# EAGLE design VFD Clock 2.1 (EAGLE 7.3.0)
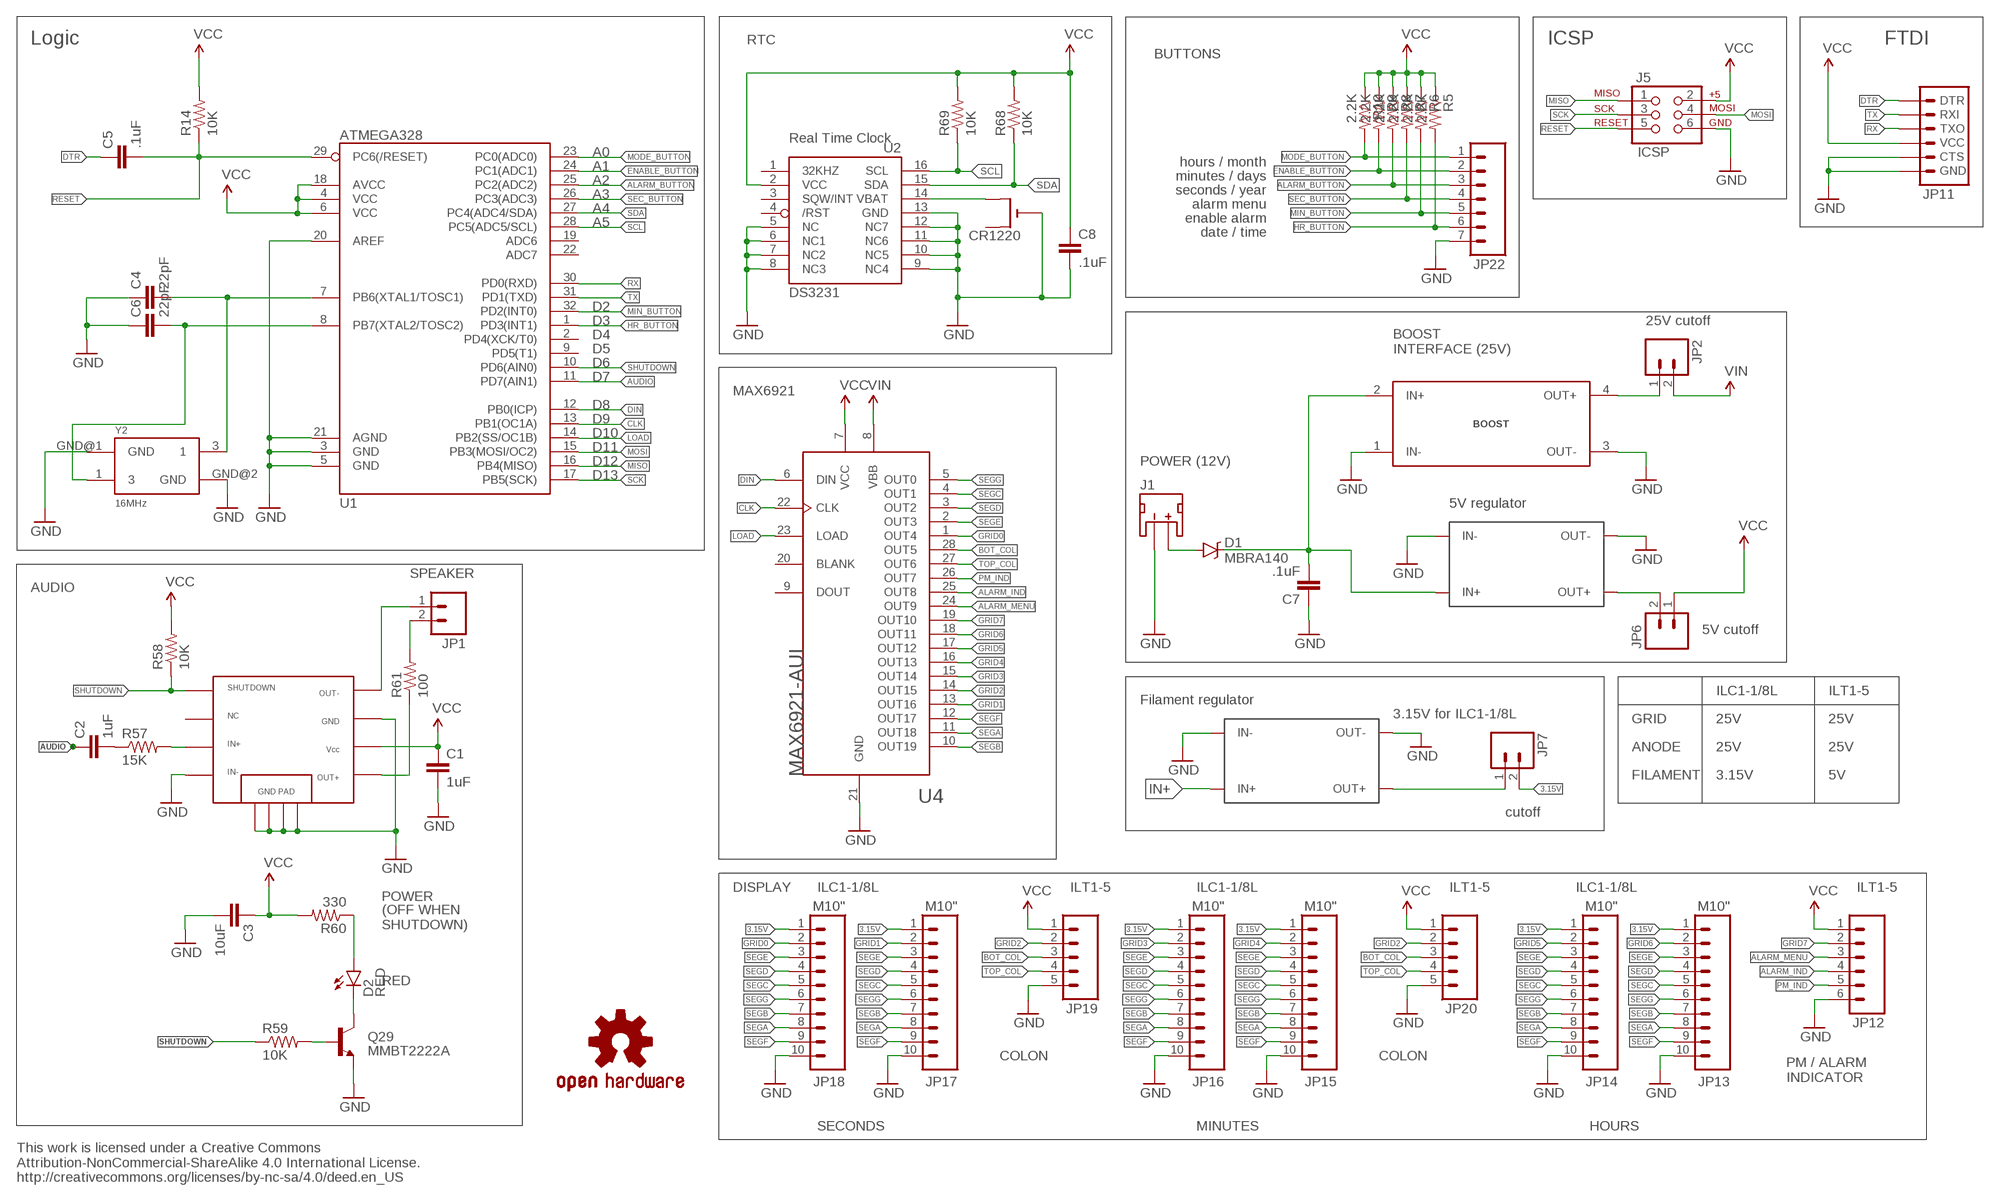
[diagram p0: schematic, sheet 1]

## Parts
3.15V  DCTODC  [DCTODC]
5V  DCTODC  [DCTODC]
C1  1uF  CAP0805  [0805]
C2  1uF  CAP0805  [0805]
C3  10uF  CAP0805  [0805]
C4  22pF  CAP0805  [0805]
C5  .1uF  CAP0805  [0805]
C6  22pF  CAP0805  [0805]
C7  .1uF  CAP0805  [0805]
C8  .1uF  CAP0805  [0805]
CR1220  CR1220SMT  [CR1220-SMD]
D1  MBRA140  [SMA-DIODE]
D2  RED  LED1206  [LED-1206]
J1  JST_2MM_MALE  [JST-2-SMD]
J5  ICSP  AVR_SPI_PRG_6PTH  [2X3]
JP1  M02PTH  [1X02]
JP2  M02PTH  [1X02]
JP6  M02PTH  [1X02]
JP7  M02PTH  [1X02]
JP11  ARDUINO_SERIAL_PROGRAMSMD  [1X06-SMD]
JP12  M06SIP  [1X06]
JP13  M10"  [1X10]
JP14  M10"  [1X10]
JP15  M10"  [1X10]
JP16  M10"  [1X10]
JP17  M10"  [1X10]
JP18  M10"  [1X10]
JP19  M05PTH  [1X05]
JP20  M05PTH  [1X05]
JP22  M07  [1X07]
Q29  MMBT2222A  TRANSISTOR_NPNSOT23-3  [SOT23-3]
R5  2.2K  RESISTOR0805-RES  [0805]
R6  2.2K  RESISTOR0805-RES  [0805]
R7  2.2K  RESISTOR0805-RES  [0805]
R8  2.2K  RESISTOR0805-RES  [0805]
R9  2.2K  RESISTOR0805-RES  [0805]
R10  2.2K  RESISTOR0805-RES  [0805]
R14  10K  RESISTOR0805-RES  [0805]
R57  15K  RESISTOR0805-RES  [0805]
R58  10K  RESISTOR0805-RES  [0805]
R59  10K  RESISTOR0805-RES  [0805]
R60  330  RESISTOR0805-RES  [0805]
R61  100  RESISTOR0805-RES  [0805]
R68  10K  RESISTOR0805-RES  [0805]
R69  10K  RESISTOR0805-RES  [0805]
U1  ATMEGA328  ATMEGA328_SMT  [TQFP32-08]
U2  DS3231  DS3231/SO  [SO16W]
U3  TPA2005  [MSOP8]
U4  MAX6921  [MAX6921]
U$2  BOOST  [BOOST]
U$7  OSHW-LOGOS  [OSHW-LOGO-S]
Y2  16MHz  OSCILLATOR5X3  [CRYSTAL-SMD-5X3]

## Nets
3.15V: JP7.2 JP13.1 JP14.1 JP15.1 JP16.1 JP17.1 JP18.1
5VOUT: 5V.OUT+ JP6.2
ALARM_BUTTON: JP22.3 R8.2 U1.25(PC2(ADC2))
ALARM_IND: JP12.4 U4.25(OUT8)
ALARM_MENU: JP12.3 U4.24(OUT9)
AUDIO: C2.1 U1.11(PD7(AIN1))
BOT_COL: JP19.3 JP20.3 U4.28(OUT5)
CLK: U1.13(PB1(OC1A)) U4.22(CLK)
DIN: U1.12(PB0(ICP)) U4.6(DIN)
DTR: C5.1 JP11.1(DTR)
ENABLE_BUTTON: JP22.2 R9.2 U1.24(PC1(ADC1))
FILAMENTOUT: 3.15V.OUT+ JP7.1
GND: 3.15V.IN- 3.15V.OUT- 5V.IN- 5V.OUT- C1.2 C3.2 C4.1 C6.1 C7.1 C8.2 CR1220.- J1.1(-) J5.6 JP11.5(CTS) JP11.6(GND) JP12.6 JP13.10 JP14.10 JP15.10 JP16.10 JP17.10 JP18.10 JP19.5 JP20.5 JP22.7 Q29.2(E) U1.3(GND) U1.5(GND) U1.20(AREF) U1.21(AGND) U2.5(NC) U2.6(NC1) U2.7(NC2) U2.8(NC3) U2.9(NC4) U2.10(NC5) U2.11(NC6) U2.12(NC7) U2.13(GND) U3.4 U3.7 U3.A U3.B U3.C U3.D U4.21(GND) U$2.1(IN-) U$2.3(OUT-) Y2.GND@1(GND) Y2.GND@2(GND)
GRID0: JP18.2 U4.1(OUT4)
GRID1: JP17.2 U4.13(OUT16)
GRID2: JP19.2 JP20.2 U4.14(OUT15)
GRID3: JP16.2 U4.15(OUT14)
GRID4: JP15.2 U4.16(OUT13)
GRID5: JP14.2 U4.17(OUT12)
GRID6: JP13.2 U4.18(OUT11)
GRID7: JP12.2 U4.19(OUT10)
HR_BUTTON: JP22.6 R5.2 U1.1(PD3(INT1))
IN+: 3.15V.IN+ 5V.IN+ C7.2 D1.C U$2.2(IN+)
IN+AMP: R57.2 U3.3
LOAD: U1.14(PB2(SS/OC1B)) U4.23(LOAD)
MIN_BUTTON: JP22.5 R6.2 U1.32(PD2(INT0))
MISO: J5.1 U1.16(PB4(MISO))
MODE_BUTTON: JP22.1 R10.2 U1.23(PC0(ADC0))
MOSI: J5.4 U1.15(PB3(MOSI/OC2))
N$1: JP2.1 U$2.4(OUT+)
N$7: CR1220.+$2(+1) U2.14(VBAT)
N$8: C6.2 U1.8(PB7(XTAL2/TOSC2)) Y2.1
N$28: JP1.2 R61.2
N$29: D2.A R60.1
N$30: C4.2 U1.7(PB6(XTAL1/TOSC1)) Y2.3
N$31: Q29.1(B) R59.2
N$33: D2.C Q29.3(C)
N$34: C2.2 R57.1
N$35: JP1.1 U3.8
N$36: R61.1 U3.5
N$39: D1.A J1.2(+)
PM_IND: JP12.5 U4.26(OUT7)
RESET: C5.2 J5.5 R14.1 U1.29(PC6(/RESET))
RX: JP11.3(TXO) U1.30(PD0(RXD))
SCK: J5.3 U1.17(PB5(SCK))
SCL: R69.1 U1.28(PC5(ADC5/SCL)) U2.16(SCL)
SDA: R68.1 U1.27(PC4(ADC4/SDA)) U2.15(SDA)
SEC_BUTTON: JP22.4 R7.2 U1.26(PC3(ADC3))
SEGA: JP13.8 JP14.8 JP15.8 JP16.8 JP17.8 JP18.8 U4.11(OUT18)
SEGB: JP13.7 JP14.7 JP15.7 JP16.7 JP17.7 JP18.7 U4.10(OUT19)
SEGC: JP13.5 JP14.5 JP15.5 JP16.5 JP17.5 JP18.5 U4.4(OUT1)
SEGD: JP13.4 JP14.4 JP15.4 JP16.4 JP17.4 JP18.4 U4.3(OUT2)
SEGE: JP13.3 JP14.3 JP15.3 JP16.3 JP17.3 JP18.3 U4.2(OUT3)
SEGF: JP13.9 JP14.9 JP15.9 JP16.9 JP17.9 JP18.9 U4.12(OUT17)
SEGG: JP13.6 JP14.6 JP15.6 JP16.6 JP17.6 JP18.6 U4.5(OUT0)
SHUTDOWN: R58.1 R59.1 U1.10(PD6(AIN0)) U3.1
TOP_COL: JP19.4 JP20.4 U4.27(OUT6)
TX: JP11.2(RXI) U1.31(PD1(TXD))
VCC: C1.1 C3.1 C8.1 J5.2 JP6.1 JP11.4(VCC) JP12.1 JP19.1 JP20.1 R5.1 R6.1 R7.1 R8.1 R9.1 R10.1 R14.2 R58.2 R60.2 R68.2 R69.2 U1.4(VCC) U1.6(VCC) U1.18(AVCC) U2.2(VCC) U3.6 U4.7(VCC)
VIN: JP2.2 U4.8(VBB)
Unconnected: CR1220.+$1(+) J1.NC1(PAD1) J1.NC2(PAD2) U1.2(PD4(XCK/T0)) U1.9(PD5(T1)) U1.19(ADC6) U1.22(ADC7) U2.1(32KHZ) U2.3(SQW/INT) U2.4(/RST) U3.NC U4.9(DOUT) U4.20(BLANK)

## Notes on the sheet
- Logic | RTC | ICSP | FTDI
- BUTTONS
- Real Time Clock
- A0 | hours / month
- A1 | minutes / days
- A2 | seconds / year
- A3 | alarm menu
- A4 | enable alarm
- A5 | date / time
- D2
- D3 | 25V cutoff
- D4
- D5
- BOOST
  INTERFACE (25V)
- D6
- D7
- MAX6921
- D8
- D9
- D10
- D11
- D12 | POWER (12V)
- D13
- 5V regulator
- SPEAKER
- AUDIO
- 5V cutoff
- ILC1-1/8L | ILT1-5
- Filament regulator
- 3.15V for ILC1-1/8L | GRID | 25V | 25V
- ANODE | 25V | 25V
- FILAMENT | 3.15V | 5V
- cutoff
- DISPLAY | ILC1-1/8L | ILT1-5 | ILC1-1/8L | ILT1-5 | ILC1-1/8L | ILT1-5
- POWER
- (OFF WHEN 
  SHUTDOWN)
- RED
- COLON | COLON
- PM / ALARM
  INDICATOR
- SECONDS | MINUTES | HOURS
- This work is licensed under a Creative Commons
  Attribution-NonCommercial-ShareAlike 4.0 International License.
  http://creativecommons.org/licenses/by-nc-sa/4.0/deed.en_US

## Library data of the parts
3.15V 5V = DC to DC:DCTODC
C1-C8 = SparkFun-Capacitors:CAP: Capacitor
CR1220 = adafruit:CR1220: CR1216/CR1220/CR1225 12mm 3V lithium coin cell Great for battery packup. Both SMT and THM holders. Note the THM package has the ground pads on both sides of the PCB so that the masks are the same - this reduces the cost
D1 = SparkFun-DiscreteSemi:MBRA140: 40V, 1A Schottky rectifier; PROD_ID: DIO-08053
D2 = SparkFun-LED:LED: LEDs
J1 = SparkFun-Connectors:JST_2MM_MALE: Mates to single-cell LiPo batteries. CONN-11443 Now with smashable polarity marks!; BTM_NEG: -; BTM_POS: +; PROD_ID: CONN-11443; TOP_NEG: -; TOP_POS: +
J5 = SparkFun:AVR_SPI_PRG_6: AVR ISP 6 Pin This is the reduced ISP connector for AVR programming. Common on Arduino. This footprint will take up less PCB space and can be used with a 10-pin to 6-pin adapter such as SKU: BOB-08508; OC_NEWARK: unknown
JP1 JP2 JP6 JP7 = SparkFun:M02: Header 2
JP11 = SparkFun-Connectors:ARDUINO_SERIAL_PROGRAM: FTDI connector footprints; PROD_ID: CONN-08971
JP12 = SparkFun-Connectors:M06: Header 6 Standard 6-pin 0.1" header. Use with straight break away headers (SKU : PRT-00116), right angle break away headers (PRT-00553), swiss pins (PRT-00743), machine pins (PRT-00117), and female headers (PRT-00115). Molex polarized connector foot print use with SKU : PRT-08094 with associated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
JP13-JP18 = SparkFun-Connectors:M10: Header 10 Standard 10-pin 0.1" header. Use with straight break away headers (SKU : PRT-00116), right angle break away headers (PRT-00553), swiss pins (PRT-00743), machine pins (PRT-00117), and female headers (PRT-00115).
JP19 JP20 = SparkFun-Connectors:M05: Header 5 Standard 5-pin 0.1" header. Use with straight break away headers (SKU : PRT-00116), right angle break away headers (PRT-00553), swiss pins (PRT-00743), machine pins (PRT-00117), and female headers (PRT-00115). Molex polarized connector foot print use with SKU : PRT-08230 with associated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
JP22 = SparkFun-Connectors:M07: Header 7 Standard 7-pin 0.1" header. Use with straight break away headers (SKU : PRT-00116), right angle break away headers (PRT-00553), swiss pins (PRT-00743), machine pins (PRT-00117), and female headers (PRT-00115). NOTES ON THE VARIANTS LOCK and LOCK_LONGPADS... This footprint was designed to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
Q29 = SparkFun:TRANSISTOR_NPN: Transistor NPN BJT configuration in SOT23 package. MMBT2222 is the common NPN we use. Double check BCE configuration again layout.
R5-R10 R14 R57-R61 R68 R69 = SparkFun-Resistors:RESISTOR: Resistor
U1 = SparkFun-DigitalIC:ATMEGA328_SMT: 32-Pin Atmega328 part Commonly used on Arduino compatible boards Available in QFP and QFN packages TQFP is IC-09069 QFN is non-stock; PROD_ID: IC-09069; VALUE: ATMEGA328P
U2 = adafruit:DS3231
U3 = TPA2005:TPA2005
U4 = MAX6921:MAX6921
U$2 = BOOST:BOOST
U$7 = SparkFun:OSHW-LOGO: Open Source Hardware Logo This logo indicates the piece of hardware it is found on incorporates a OSHW license and/or adheres to the definition of open source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
Y2 = SparkFun-FreqCtrl:OSCILLATOR: Generic 5x3 and 7x5 oscillators

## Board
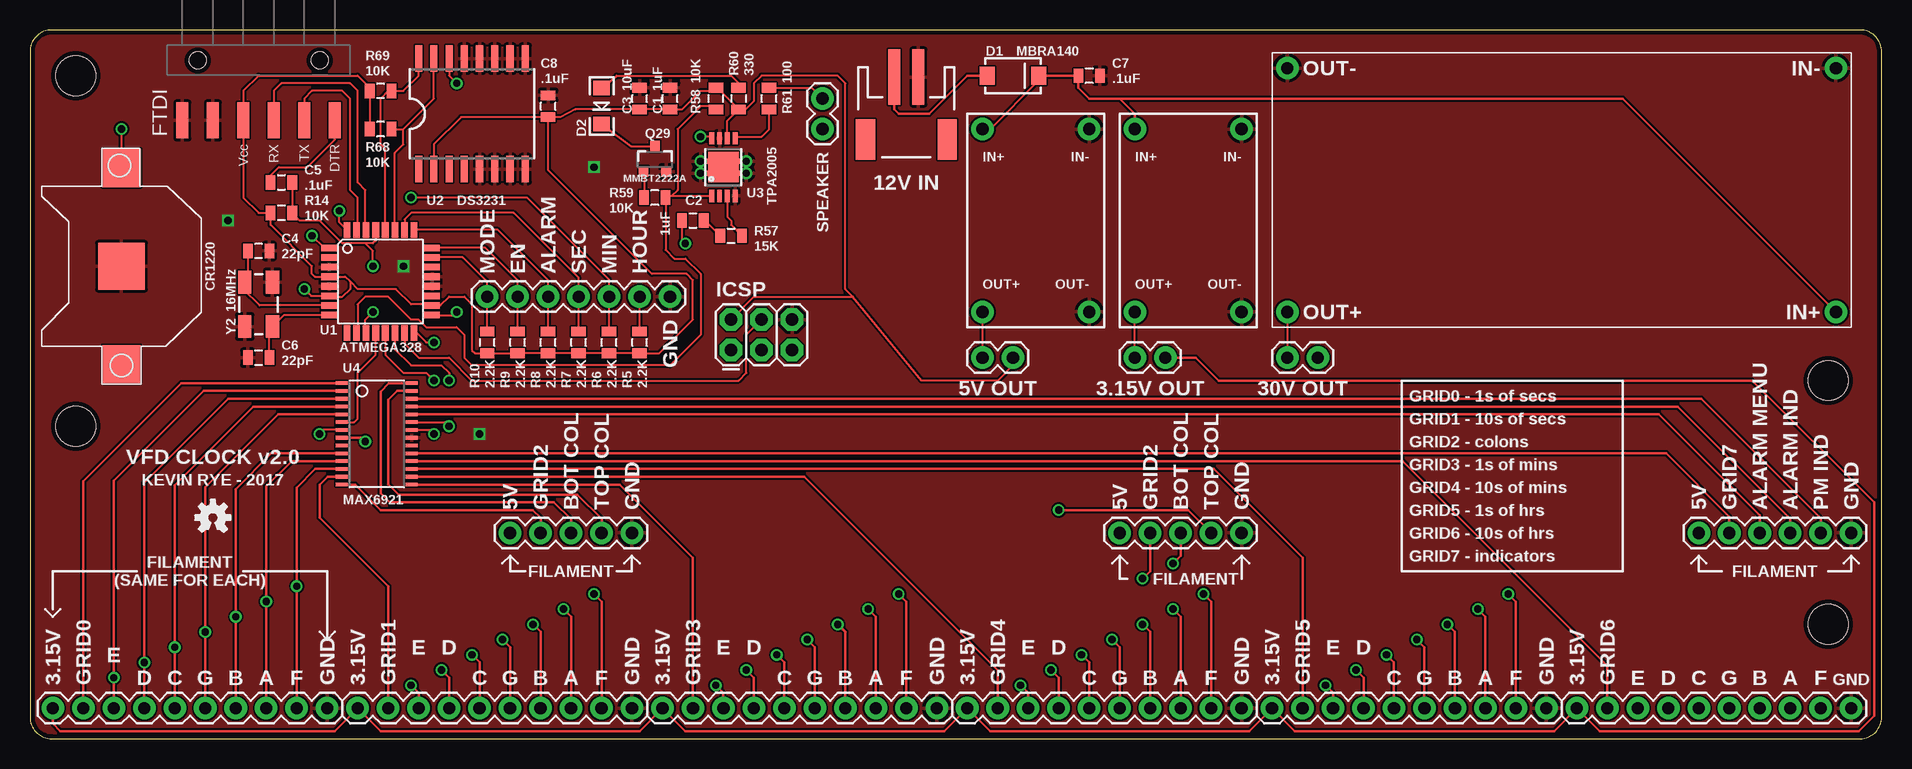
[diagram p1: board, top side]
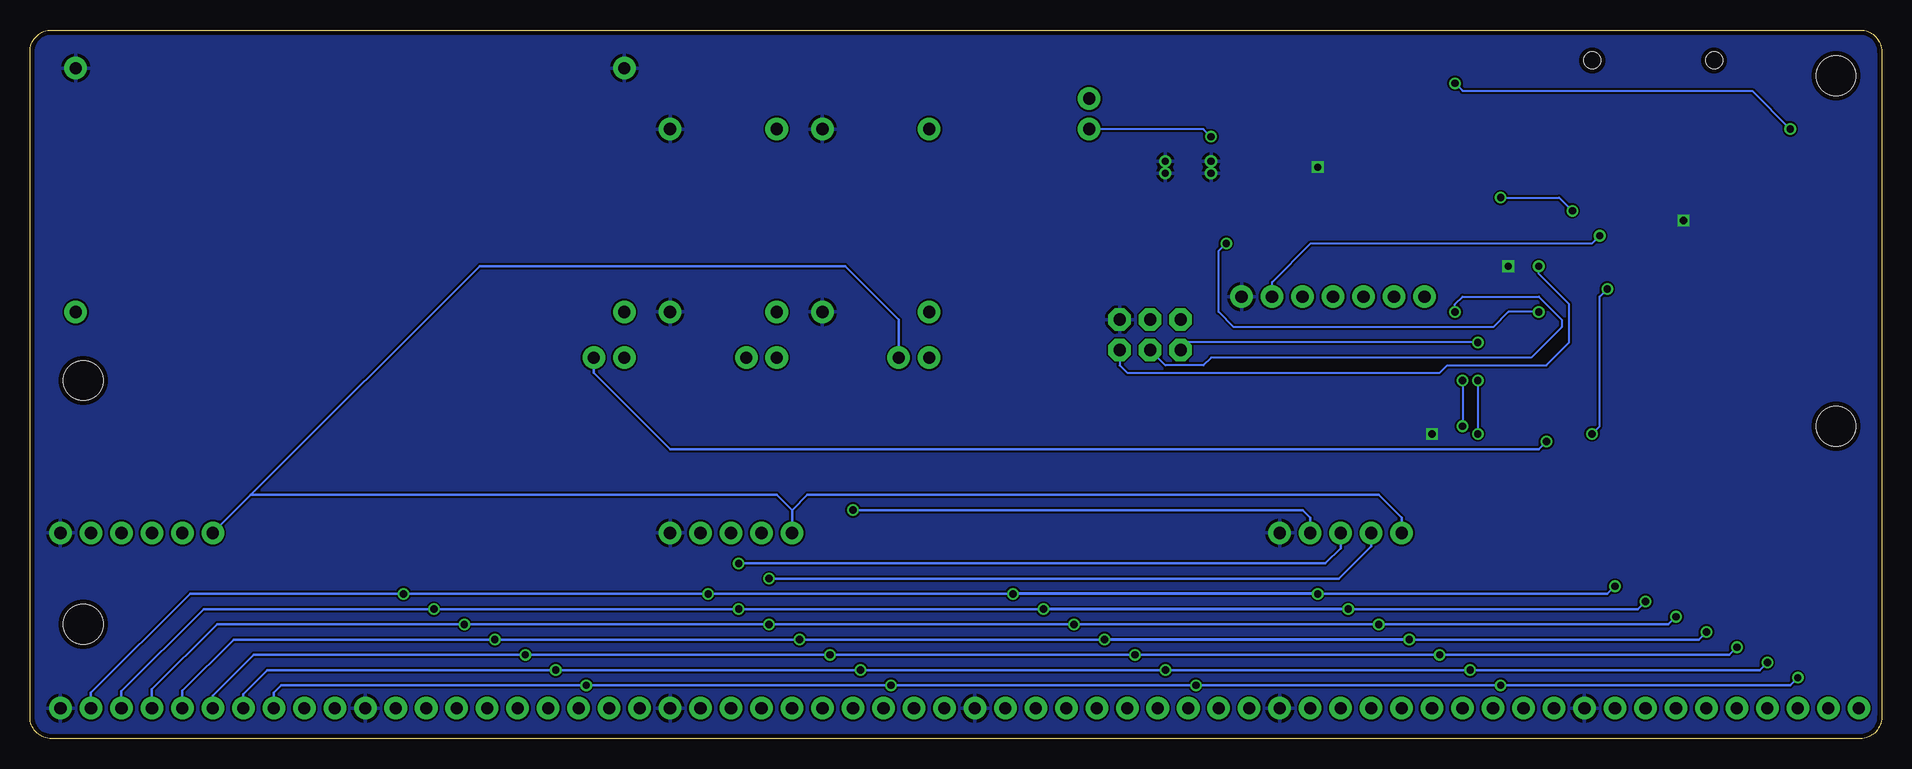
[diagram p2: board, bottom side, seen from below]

Size 154.31 x 59.05 mm. Coordinates in mm from the lower left corner, seen from the top.
Outline: 152.51,59.05 1.8,59.05 arc90 0,57.26 0,1.8 arc90 1.8,0 152.51,0 arc90 154.31,1.8 154.31,57.26 arc90 152.51,59.05
Copper layers (1*16): Top 0.0356mm / dielectric 1.5011mm / Bottom 0.0356mm
Design rules "oshpark-2layer": minimum track width 6mil, minimum drill 13mil, track to track 6mil, track to pad 6mil, pad to pad 6mil, via to via 6mil, smd to smd 6mil, copper to edge 15mil, drill to drill 6mil, minimum pad ring 7mil, minimum via ring 7mil, stop-mask expansion 2.5mil, vias tented up to drill 0mil, thermal gap 10mil

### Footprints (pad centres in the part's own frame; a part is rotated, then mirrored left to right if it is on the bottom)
DCTODC = drill 1.016 pad 1.88: IN+ 10.16,1.27; IN- 1.27,1.27; OUT+ 10.16,16.51; OUT- 1.27,16.51
0805 = smd 0.8 x 1.2: 1 -0.9,0; 2 0.9,0
CR1220-SMD = smd 3.2 x 3.2: +$1 -8.2,0; +$2 8.2,0 | smd 3.9 x 3.9: - 0,0
SMA-DIODE = smd 1.27 x 1.47: A -2.15,0; C 2.15,0
LED-1206 = smd 1.2 x 1.4: A -1.5,0; C 1.5,0
JST-2-SMD = smd 1 x 4.6: 1 -1,-3.7; 2 1,-3.7 | smd 1.6 x 3.4: NC1 -3.4,1.5; NC2 3.4,1.5
2X3 = drill 1.016 pad 1.88 octagon: 1 0,0; 2 0,2.54; 3 2.54,0; 4 2.54,2.54; 5 5.08,0; 6 5.08,2.54
1X02 = drill 1.016 pad 1.88: 1 0,0; 2 2.54,0
1X06-SMD = smd 1 x 3: 1 -6.35,5; 2 -3.81,5; 3 -1.27,5; 4 1.27,5; 5 3.81,5; 6 6.35,5 | hole 1.4: -5.08,0; 5.08,0
1X06 = drill 1.016 pad 1.88: 1 0,0; 2 2.54,0; 3 5.08,0; 4 7.62,0; 5 10.16,0; 6 12.7,0
1X10 = drill 1.016 pad 1.88: 1 0,0; 2 2.54,0; 3 5.08,0; 4 7.62,0; 5 10.16,0; 6 12.7,0; 7 15.24,0; 8 17.78,0; 9 20.32,0; 10 22.86,0
1X05 = drill 1.016 pad 1.88: 1 0,0; 2 2.54,0; 3 5.08,0; 4 7.62,0; 5 10.16,0
1X07 = drill 1.016 pad 1.88: 1 0,0; 2 2.54,0; 3 5.08,0; 4 7.62,0; 5 10.16,0; 6 12.7,0; 7 15.24,0
SOT23-3 = smd 0.8 x 0.9: 1 -0.95,-1; 2 0.95,-1; 3 0,1.1
TQFP32-08 = smd 1.27 x 0.559: 1 -4.293,2.8; 2 -4.293,2; 3 -4.293,1.2; 4 -4.293,0.4; 5 -4.293,-0.4; 6 -4.293,-1.2; 7 -4.293,-2; 8 -4.293,-2.8; 17 4.293,-2.8; 18 4.293,-2; 19 4.293,-1.2; 20 4.293,-0.4; 21 4.293,0.4; 22 4.293,1.2; 23 4.293,2; 24 4.293,2.8 | smd 0.559 x 1.27: 9 -2.8,-4.293; 10 -2,-4.293; 11 -1.2,-4.293; 12 -0.4,-4.293; 13 0.4,-4.293; 14 1.2,-4.293; 15 2,-4.293; 16 2.8,-4.293; 25 2.8,4.293; 26 2,4.293; 27 1.2,4.293; 28 0.4,4.293; 29 -0.4,4.293; 30 -1.2,4.293; 31 -2,4.293; 32 -2.8,4.293
SO16W = smd 0.6 x 2.2: 1 -4.445,-4.6; 2 -3.175,-4.6; 3 -1.905,-4.6; 4 -0.635,-4.6; 5 0.635,-4.6; 6 1.905,-4.6; 7 3.175,-4.6; 8 4.445,-4.6; 9 4.445,4.6; 10 3.175,4.6; 11 1.905,4.6; 12 0.635,4.6; 13 -0.635,4.6; 14 -1.905,4.6; 15 -3.175,4.6; 16 -4.445,4.6
MSOP8 = smd 0.41 x 1.02: 1 -0.975,-2.4; 3 0.325,-2.4; 4 0.975,-2.4; 5 0.975,2.4; 6 0.325,2.4; 7 -0.325,2.4; 8 -0.975,2.4; NC -0.325,-2.4 | smd 1.02 x 0.41: 2 -1.13,0.5; 9 -1.13,-0.5; 10 1.13,-0.5; 11 1.13,0.5 | drill 0.61 pad 1.016: A -1.9,-0.5; B 1.91,-0.5; C 1.91,0.5; D -1.9,0.5 | smd 2.54 x 1.27: GND 0,0.635; GND1 0,0.635; GND* 0,-0.635
MAX6921 = smd 0.991 x 0.305: 1 -0.695,8.67; 2 -0.695,8.02; 3 -0.695,7.37; 4 -0.695,6.72; 5 -0.695,6.07; 6 -0.695,5.42; 7 -0.695,4.77; 8 -0.695,4.12; 9 -0.695,3.47; 10 -0.695,2.82; 11 -0.695,2.17; 12 -0.695,1.52; 13 -0.695,0.87; 14 -0.695,0.22; 15 5.14,0.22; 16 5.14,0.87; 17 5.14,1.52; 18 5.14,2.17; 19 5.14,2.82; 20 5.14,3.47; 21 5.14,4.12; 22 5.14,4.77; 23 5.14,5.42; 24 5.14,6.07; 25 5.14,6.72; 26 5.14,7.37; 27 5.14,8.02; 28 5.14,8.67
BOOST = drill 1.016 pad 1.88: 1 1.27,1.27; 2 1.27,21.59; 3 46.99,1.27; 4 46.99,21.59
STAND-OFF = hole 3.302: 0,0
CRYSTAL-SMD-5X3 = smd 1.9 x 1.1: 1 -1.85,-1.15; 3 1.85,1.15; GND@1 -1.85,1.15; GND@2 1.85,-1.15

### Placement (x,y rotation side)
3.15V  102.23,52.07 180 top
5V  89.53,52.07 180 top
C1  53.34,53.34 90 top
C2  55.24,43.18 0 top
C3  50.8,53.34 90 top
C4  19.05,40.64 180 top
C5  20.95,46.36 0 top
C6  19.05,31.75 0 top
C7  88.27,55.25 180 top
C8  43.18,52.71 90 top
CR1220  7.62,39.37 90 top
D1  81.92,55.25 0 top
D2  47.62,52.71 270 top
J1  73.03,51.44 180 top
J5  58.42,32.39 0 top
JP1  66.04,50.8 90 top
JP2  104.78,31.75 0 top
JP6  81.92,31.75 180 top
JP7  92.08,31.75 0 top
JP11  19.05,56.52 180 top
JP12  139.06,17.14 0 top
JP13  128.91,2.54 0 top
JP14  103.5,2.54 0 top
JP15  78.11,2.54 0 top
JP16  52.7,2.54 0 top
JP17  27.3,2.54 0 top
JP18  1.91,2.54 0 top
JP19  40.01,17.14 0 top
JP20  90.81,17.14 0 top
JP22  38.1,36.83 0 top
Q29  52.07,48.26 0 top
R5  50.8,33.02 90 top
R6  48.26,33.02 90 top
R7  45.72,33.02 90 top
R8  43.18,33.02 90 top
R9  40.64,33.02 90 top
R10  38.1,33.02 90 top
R14  20.95,43.82 180 top
R57  58.42,41.91 0 top
R58  57.15,53.34 90 top
R59  52.07,45.09 180 top
R60  59.05,53.34 270 top
R61  61.59,53.34 90 top
R68  29.21,50.8 180 top
R69  29.21,53.98 180 top
U1  29.21,38.1 0 top
U2  36.83,52.07 0 top
U3  57.78,47.62 0 top
U4  26.67,20.95 0 top
U$2  151.76,57.15 180 top
U$3  [STAND-OFF]  3.81,55.25 0 top
U$4  [STAND-OFF]  149.86,29.84 0 top
U$5  [STAND-OFF]  149.86,9.53 0 top
U$6  [STAND-OFF]  3.81,26.04 0 top
U$7  15.24,18.41 0 top
Y2  19.05,36.2 90 top

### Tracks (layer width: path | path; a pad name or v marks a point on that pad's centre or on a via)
3.15V
  Top 0.229: JP18.1 1.91,1.27 2.54,0.64 25.4,0.64 JP17.1 29.21,0.64 50.8,0.64 JP16.1 54.61,0.64 76.2,0.64 JP15.1 80.01,0.64 101.6,0.64 JP14.1 105.41,0.64 127,0.64 JP13.1 130.81,0.64 152.4,0.64 153.67,1.91 153.67,19.68 143.51,29.84 99.06,29.84 97.16,31.75 JP7.2
5VOUT
  Top 0.178: JP6.2 5V.OUT+
ALARM_BUTTON
  Top 0.178: U1.25 38.99,42.39 43.18,38.2 JP22.3 R8.2
ALARM_IND
  Top 0.229: U4.25 137.33,27.67 146.69,18.32 JP12.4
ALARM_MENU
  Top 0.229: U4.24 135.75,27.02 144.15,18.63 JP12.3
AUDIO  (via drill 0.61)
  Top 0.178: U1.11 27.94,33.88 27.94,34.93 v28.57,35.56 | v54.61,41.27 54.34,41.54 C2.1
  Bottom 0.178: v28.57,35.56 31.11,35.56 32.38,34.29 53.98,34.29 55.24,35.56 55.24,40.64 v54.61,41.27
BOT_COL  (via drill 0.61)
  Top 0.229: U4.28 29.91,29.62 29.21,28.92 29.21,20.47 30,19.68 43.66,19.68 45.09,18.26 JP19.3 | v95.25,14.61 95.89,15.24 JP20.3
  Bottom 0.229: JP19.3 45.09,15.88 46.35,14.61 v95.25,14.61
CLK  (via drill 0.61)
  Top 0.178: U4.22 33.33,25.72 v33.66,25.4 | U1.13 29.61,31.98 31.11,30.48 33.02,30.48 v33.66,29.84
  Bottom 0.178: v33.66,29.84 v33.66,25.4
DIN
  Top 0.178: U4.6 27.01,26.38 27.3,26.67 27.3,30.48 28.81,31.98 U1.12
DTR
  Top 0.178: JP11.1 25.4,49.91 23.11,47.62 20.74,47.62 20.05,46.94 C5.1
ENABLE_BUTTON
  Top 0.178: U1.24 37.95,40.9 40.64,38.21 JP22.2 R9.2
FILAMENTOUT
  Top 0.178: JP7.1 3.15V.OUT+
GND  (via drill 0.61)
  other vias: 46.99,47.62 31.11,39.37 37.47,25.4 16.51,43.18
  pour Top: -1.27,60.33 155.57,60.33 155.57,-1.27 -1.27,-1.91
  pour Bottom: -0.64,59.69 154.94,59.69 154.94,-0.64 -0.64,-0.64
GRID0
  Top 0.229: U4.1 12.61,29.62 4.45,21.46 JP18.2
GRID1
  Top 0.229: U4.13 24.81,21.82 24.13,21.15 24.13,18.41 29.84,12.7 JP17.2
GRID2  (via drill 0.61)
  Top 0.229: JP19.2 42.55,18.41 41.91,19.05 29.21,19.05 27.09,21.17 U4.14 | v92.71,13.34 93.34,13.97 JP20.2
  Bottom 0.229: JP19.2 42.55,16.03 45.24,13.34 v92.71,13.34
GRID3
  Top 0.229: U4.15 49.13,21.17 55.24,15.06 JP16.2
GRID4
  Top 0.229: U4.16 64.5,21.82 80.64,5.69 JP15.2
GRID5
  Top 0.229: U4.17 98.65,22.47 106.05,15.08 JP14.2
GRID6
  Top 0.229: JP13.2 131.44,6.07 114.39,23.12 U4.18
GRID7
  Top 0.229: U4.19 136.34,23.77 141.6,18.51 JP12.2
HR_BUTTON  (via drill 0.61)
  Top 0.178: v23.5,41.91 24.5,40.9 U1.1 | R5.2 JP22.6
  Bottom 0.178: JP22.6 50.8,38.04 47.56,41.27 24.13,41.27 v23.5,41.91
IN+
  Top 0.178: 84.06,54.86 D1.C
  Top 0.229: D1.C C7.2 87.36,54.24 88.27,53.34 90.81,53.34 | 5V.IN+ 80.01,50.8 84.06,54.86 | 90.81,53.34 132.72,53.34 U$2.2 | 3.15V.IN+ 92.08,52.07 90.81,53.34
IN+AMP
  Top 0.178: U3.3 58.11,43.49 58.42,43.18 58.42,42.81 R57.2
LOAD  (via drill 0.61)
  Top 0.178: U4.23 34.59,26.38 v34.92,26.04 | U1.14 30.41,32.46 31.75,31.11 34.29,31.11 34.92,30.48 v34.92,29.84
  Bottom 0.178: v34.92,29.84 v34.92,26.04
MIN_BUTTON  (via drill 0.61)
  Top 0.178: v31.75,45.09 41.42,45.09 48.26,38.25 JP22.5 R6.2 | U1.32 25.77,43.03 v25.77,43.99
  Bottom 0.178: v31.75,45.09 26.87,45.09 v25.77,43.99
MISO  (via drill 0.61)
  Top 0.178: U1.16 32.23,33.81 33.02,33.02 v33.66,33.02
  Bottom 0.178: v33.66,33.02 57.78,33.02 J5.1
MODE_BUTTON
  Top 0.178: U1.23 36.06,40.1 38.1,38.06 JP22.1 R10.2
MOSI
  Top 0.178: U1.15 31.21,32.93 32.38,31.75 34.92,31.75 36.83,29.84 59.05,29.84 59.69,30.48 59.69,33.66 J5.4
N$1
  Top 0.178: U$2.4 JP2.1
N$7  (via drill 0.61)
  Top 0.178: U2.14 34.92,55.25 v35.56,54.61 | v7.62,50.8 CR1220.+$2
  Bottom 0.178: v35.56,54.61 34.92,53.98 10.79,53.98 v7.62,50.8
N$8
  Top 0.178: U1.8 21.16,35.3 Y2.1 19.95,34.09 C6.2
N$28
  Top 0.178: R61.2 65.14,54.24 JP1.2
N$29
  Top 0.178: D2.A 48.9,55.25 58.42,55.25 59.05,54.61 R60.1
N$30
  Top 0.178: U1.7 19.14,36.1 17.78,37.47 17.78,37.93 Y2.3 18.15,38.3 C4.2
N$31
  Top 0.178: Q29.1 51.17,47.21 R59.2
N$33
  Top 0.178: D2.C 50.1,49.36 Q29.3
N$34
  Top 0.178: R57.1 56.25,43.18 C2.2
N$35  (via drill 0.61)
  Top 0.178: U3.8 56.67,50.16 v55.88,50.16
  Bottom 0.178: v55.88,50.16 56.52,50.8 JP1.1
N$36
  Top 0.178: U3.5 58.76,50.24 58.84,50.16 60.96,50.16 61.59,50.8 R61.1
N$39
  Top 0.178: 79.77,55 D1.A
  Top 0.229: J1.2 72.03,52.44 72.39,52.07 74.93,52.07 78.11,55.25 D1.A
PM_IND
  Top 0.229: U4.26 139.26,28.32 149.22,18.36 JP12.5
RESET  (via drill 0.61)
  Top 0.178: C5.2 R14.1 22.49,43.18 24.13,43.18 26.04,41.27 27.94,41.27 | U1.29 28.81,41.51 28.57,41.27 27.94,41.27 | v28.57,39.37 28.57,40.64 27.94,41.27
  Bottom 0.178: J5.5 63.5,31.11 62.87,30.48 36.83,30.48 36.2,31.11 27.94,31.11 26.04,33.02 26.04,36.2 28.57,38.73 v28.57,39.37
RX
  Top 0.178: U1.30 27.94,42.46 27.94,45.72 27.3,46.36 27.3,53.98 26.67,54.61 20.95,54.61 20.32,53.98 JP11.3
SCK  (via drill 0.61)
  Top 0.178: U1.17 35.3,35.3 v35.56,35.56
  Bottom 0.178: v35.56,35.56 35.56,36.2 34.92,36.83 28.57,36.83 26.67,34.93 26.67,34.29 29.21,31.75 55.88,31.75 56.52,31.11 59.69,31.11 J5.3
SCL
  Top 0.178: U2.16 32.38,55.25 31.11,53.98 R69.1 29.84,53.98 29.21,53.34 29.21,49.53 29.61,49.13 U1.28
SDA
  Top 0.178: R68.1 31.11,50.8 | 31.11,50.8 33.66,53.34 U2.15 | U1.27 30.41,48.83 31.11,49.53 31.11,50.8
SEC_BUTTON
  Top 0.178: U1.26 31.21,43.27 31.75,43.82 40.3,43.82 45.72,38.39 JP22.4 R7.2
SEGA  (via drill 0.61)
  Top 0.229: U4.11 21.79,23.12 19.68,21.02 v19.68,11.43 JP18.8 | v44.45,10.79 45.09,10.16 JP17.8 | v69.85,10.79 70.48,10.16 JP16.8 | v95.25,10.79 95.89,10.16 JP15.8 | v120.65,10.79 121.28,10.16 JP14.8
  Bottom 0.229: v44.45,10.79 20.32,10.79 v19.68,11.43 | v69.85,10.79 v95.25,10.79 v120.65,10.79 139.85,10.79 146.69,3.96 JP13.8
  Bottom 0.254: v44.45,10.79 v69.85,10.79
SEGB  (via drill 0.61)
  Top 0.229: U4.10 20.12,23.77 17.14,20.8 v17.14,10.16 JP18.7 | JP16.7 67.94,8.89 | v41.91,9.53 42.55,8.89 JP17.7 | v92.71,9.53 93.34,8.89 JP15.7 | v118.11,9.53 118.75,8.89 JP14.7
  Top 0.254: 67.94,8.89 v67.31,9.53
  Bottom 0.229: JP13.7 144.15,4.1 138.72,9.53 v118.11,9.53 v92.71,9.53 v67.31,9.53 v41.91,9.53 17.78,9.53 v17.14,10.16
SEGC  (via drill 0.61)
  Top 0.229: U4.4 18.62,27.67 12.06,21.12 v12.06,7.62 JP18.5 | v36.83,6.99 37.47,6.35 JP17.5 | v62.23,6.99 62.87,6.35 JP16.5 | v87.63,6.99 88.27,6.35 JP15.5 | v113.03,6.99 113.67,6.35 JP14.5
  Bottom 0.229: JP13.5 139.06,3.57 135.65,6.99 v113.03,6.99 v87.63,6.99 v62.23,6.99 v36.83,6.99 12.7,6.99 v12.06,7.62
SEGD  (via drill 0.61)
  Top 0.229: U4.3 16.54,28.32 9.53,21.31 v9.53,6.35 JP18.4 | v34.29,5.71 34.92,5.08 JP17.4 | v59.69,5.71 60.33,5.08 JP16.4 | v85.09,5.71 85.72,5.08 JP15.4 | v110.49,5.71 111.12,5.08 JP14.4
  Bottom 0.229: JP13.4 136.53,3.71 134.52,5.71 v110.49,5.71 v85.09,5.71 v59.69,5.71 v34.29,5.71 10.16,5.71 v9.53,6.35
SEGE  (via drill 0.61)
  Top 0.229: U4.2 14.48,28.97 6.99,21.48 v6.99,5.08 JP18.3 | JP17.3 32.38,3.81 v31.75,4.45 | v57.15,4.45 57.78,3.81 JP16.3 | v82.55,4.45 83.19,3.81 JP15.3 | v107.95,4.45 108.58,3.81 JP14.3
  Bottom 0.229: JP13.3 133.99,3.81 133.35,4.45 v107.95,4.45 v82.55,4.45 v57.15,4.45 v31.75,4.45 7.62,4.45 v6.99,5.08
SEGF  (via drill 0.61)
  Top 0.229: U4.12 23.77,22.47 22.23,20.93 v22.23,12.7 JP18.9 | v46.99,12.06 47.62,11.43 JP17.9 | v72.39,12.06 73.03,11.43 JP16.9 | v97.79,12.06 98.42,11.43 JP15.9 | v123.19,12.06 123.83,11.43 JP14.9
  Bottom 0.229: v46.99,12.06 22.86,12.06 v22.23,12.7 | v72.39,12.06 v97.79,12.06 v123.19,12.06 140.97,12.06 149.22,3.81 JP13.9
  Bottom 0.254: v46.99,12.06 v72.39,12.06
SEGG  (via drill 0.61)
  Top 0.229: U4.5 20.7,27.02 14.61,20.93 v14.61,8.89 JP18.6 | v39.37,8.26 40.01,7.62 JP17.6 | v64.77,8.26 65.41,7.62 JP16.6 | v90.17,8.26 90.81,7.62 JP15.6 | v115.57,8.26 116.2,7.62 JP14.6
  Bottom 0.229: v39.37,8.26 15.24,8.26 v14.61,8.89 | v64.77,8.26 v90.17,8.26 v115.57,8.26 137.34,8.26 141.6,4 JP13.6
  Bottom 0.254: v39.37,8.26 v64.77,8.26
SHUTDOWN
  Top 0.178: 53.48,45.23 53.11,45.23 R59.1 52.97,40.74 53.7,40.01 54.61,40.01 55.88,38.73 55.88,33.66 53.34,31.11 36.83,31.11 36.2,31.75 36.2,33.66 35.56,34.29 33.02,34.29 32.38,34.93 31.75,34.93 29.84,36.83 27.94,36.83 27.3,36.2 27.3,33.9 U1.10 | 53.48,45.23 U3.1 | 53.48,45.23 53.98,45.72 53.98,50.8 55.88,52.71 56.88,52.71 R58.1
TOP_COL  (via drill 0.61)
  Top 0.229: U4.27 30.59,28.97 29.84,28.22 29.84,21.22 30.74,20.32 45.62,20.32 47.62,18.31 JP19.4 | v85.72,19.05 96.52,19.05 JP20.4
  Bottom 0.229: JP19.4 47.62,18.41 48.26,19.05 v85.72,19.05
TX
  Top 0.178: U1.31 27.3,42.49 27.3,45.09 26.67,45.72 26.67,53.34 26.04,53.98 23.5,53.98 22.86,53.34 JP11.2
VCC  (via drill 0.61)
  Top 0.178: C8.1 35.93,51.8 33.66,49.53 U2.2 | 26.67,38.1 26.27,38.5 U1.4 23.73,38.5 23.5,38.73 23.5,39.37 20.05,42.81 R14.2 19.05,43.82 17.78,45.09 JP11.4 17.78,53.98 19.05,55.25 27.3,55.25 28.31,54.24 R69.2 R68.2 | 26.67,38.1 26.67,37.47 26.04,36.83 24.99,36.83 U1.6 23.43,36.9 v22.86,37.47 | C8.1 43.18,47.38 51.82,38.73 54.73,38.73 55.24,38.22 55.24,34.93 52.44,32.12 R5.1 R6.1 R7.1 R8.1 R9.1 R10.1 37.09,32.12 36.83,32.39 36.83,36.2 36.2,36.83 34.92,36.83 34.2,36.1 U1.18 33.41,36.2 31.75,36.2 30.48,37.47 27.3,37.47 26.67,38.1 | R60.2 57.26,54.24 R58.2 56.88,53.98 55.88,53.98 54.34,52.44 C1.1 C3.1 45.45,52.44 44.19,51.8 C8.1 | U3.6 58.11,51.5 R60.2 | U4.7 24.45,25.72 v24.13,25.4 | 68.58,36.83 74.3,29.84 80.64,29.84 81.92,31.11 JP6.1 | J5.2 60.33,36.83 68.58,36.83 | 68.58,36.83 67.94,37.47 67.94,54.61 67.31,55.25 60.96,55.25 60.33,54.61 60.33,53.13 59.64,52.44 R60.2
  Bottom 0.178: v24.13,25.4 23.5,26.04 23.5,36.83 v22.86,37.47
  Bottom 0.229: JP19.1 40.01,18.41 41.91,20.32 89.53,20.32 90.81,19.05 | 90.81,19.05 92.08,20.32 135.89,20.32 | 135.89,20.32 JP12.1 | 90.81,19.05 JP20.1 | JP6.1 81.92,34.93 86.36,39.37 116.84,39.37 135.89,20.32
VIN  (via drill 0.61)
  Top 0.229: U4.8 27.63,25.07 v27.94,24.76
  Bottom 0.229: v27.94,24.76 28.57,24.13 99.06,24.13 100.97,24.13 107.31,30.48 JP2.2

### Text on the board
Unrouted: This work is licensed under a Creative Commons Attribution-NonCommercial-ShareAlike 4.0 International License. / http://creativecommons.org/licenses/by-nc-sa/4.0/deed.en_US
tNames: FTDI | Vcc | RX | TX | DTR | SPEAKER | 12V IN | MODE | EN | ALARM | SEC | MIN | HOUR | GND | 5V OUT | 3.15V OUT | 30V OUT | GRID0 - 1s of secs | GRID1 - 10s of secs | GRID2 - colons | VFD CLOCK v2.0 | GRID3 - 1s of mins | KEVIN RYE - 2017 | GRID4 - 10s of mins | 5V | GRID2 | BOT COL | TOP COL | GND | 5V | GRID2 | BOT COL | TOP COL | GND | GRID5 - 1s of hrs | 5V | GRID7 | ALARM MENU | ALARM IND | PM IND | GND | GRID6 - 10s of hrs | GRID7 - indicators | FILAMENT / (SAME FOR EACH) | FILAMENT | FILAMENT | FILAMENT | E | D | E | D | E | D | E | D | E | 3.15V | GRID0 | D | C | G | B | A | F | GND | 3.15V | GRID1 | C | G | B | A | F | GND | 3.15V | GRID3 | C | G | B | A | F | GND | 3.15V | GRID4 | C | G | B | A | F | GND | 3.15V | GRID5 | C | G | B | A | F | GND | 3.15V | GRID6 | E | D | C | G | B | A | F | GND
